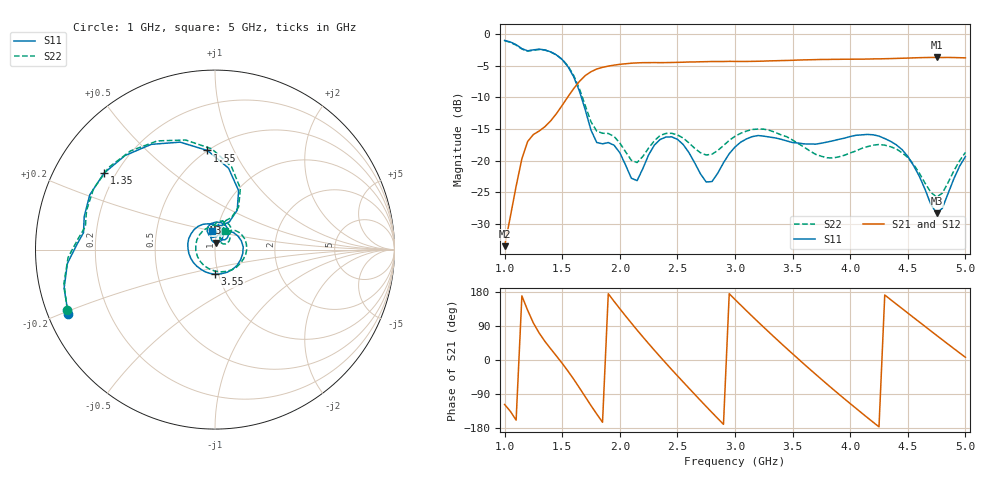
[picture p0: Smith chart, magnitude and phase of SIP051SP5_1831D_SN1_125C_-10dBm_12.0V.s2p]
# GHz  S  dB  R  50
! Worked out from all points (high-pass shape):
!   81 points, 1 GHz to 5 GHz, reference 50 ohm
!   highest |S21| = -3.67 dB at 4.75 GHz (marker M1); lowest = -33.5 dB at 1 GHz (marker M2)
!   |S21| within 3 dB of the highest: 1.693 GHz to end of sweep
!   lowest |S11| = -28.3 dB at 4.75 GHz (marker M3), VSWR 1.08, Z = 50.3 + j3.84 ohm
!   |S11| at or under -10 dB: 1.667 GHz to end of sweep
!   |S22| runs from -25.8 to -1.0 dB; largest |S21 - S12| = 0.0015
!   S11 on the Smith chart (normalised r, x): 1 GHz: 0.06, -0.21; 1.35 GHz: 0.16, +0.30; 1.55 GHz: 0.50, +0.79; 3.55 GHz: 0.97, -0.27; 5 GHz: 0.95, +0.20
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1  -0.99 -156.4  -33.53 -117.4  -33.47 -117.3  -1.02 -157.9
1.2  -2.63 172.7  -16.97 131.2  -16.97 131.2  -2.69 169.9
1.35  -2.49 145.5  -14.63 49.1  -14.63 49.2  -2.51 142.3
1.55  -5.13 94.3  -9.89 -29.3  -9.89 -29.3  -5.02 91.7
1.7  -11.96 60.6  -6.55 -97.0  -6.56 -96.9  -11.29 61.1
1.9  -17.14 82.8  -5.05 174.9  -5.04 175.0  -15.71 74.7
2.1  -22.79 83.3  -4.59 97.5  -4.58 97.6  -19.95 73.8
2.35  -16.66 98.5  -4.50 8.6  -4.49 8.6  -16.02 83.2
2.5  -16.62 66.5  -4.45 -41.6  -4.45 -41.6  -15.93 60.2
2.65  -20.35 43.9  -4.39 -90.6  -4.38 -90.5  -18.05 47.1
2.85  -22.00 70.6  -4.32 -154.2  -4.33 -154.2  -18.40 54.3
3  -17.85 53.2  -4.31 159.7  -4.30 159.7  -16.15 42.8
3.25  -16.13 -7.8  -4.25 86.3  -4.25 86.3  -15.02 1.2
3.55  -17.21 -89.4  -4.09 2.6  -4.08 2.6  -17.32 -63.1
3.7  -17.39 -126.4  -4.02 -37.7  -4.02 -37.7  -19.01 -107.3
3.85  -16.87 -160.1  -3.97 -76.9  -3.97 -76.9  -19.58 -158.2
4  -16.19 167.6  -3.96 -115.0  -3.96 -115.0  -18.79 151.0
4.2  -15.92 125.7  -3.91 -164.4  -3.92 -164.3  -17.55 95.9
4.35  -16.94 95.5  -3.86 159.6  -3.86 159.6  -17.80 63.9
4.55  -20.78 62.1  -3.74 112.0  -3.75 112.1  -20.60 31.6
4.75  -28.32 82.7  -3.67 65.0  -3.68 65.0  -25.77 45.3
5  -19.37 98.8  -3.74 7.2  -3.75 7.1  -18.71 61.0
